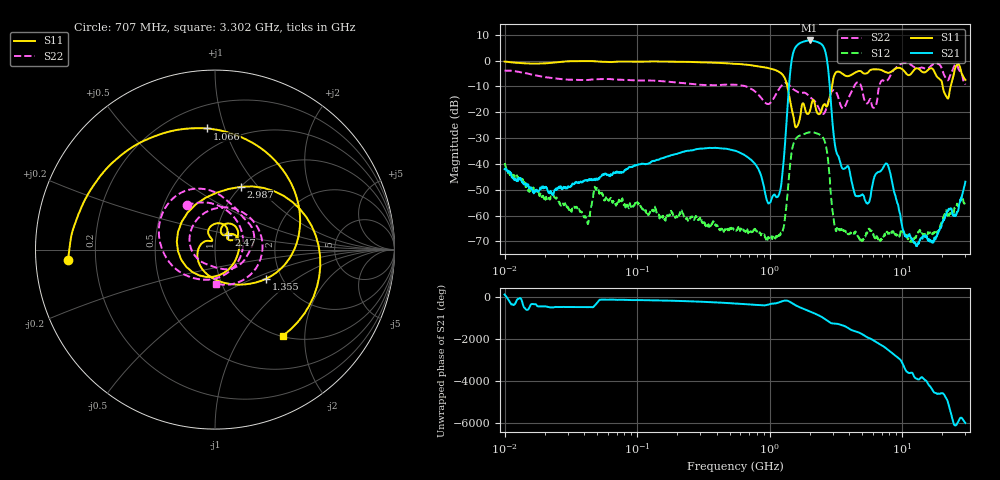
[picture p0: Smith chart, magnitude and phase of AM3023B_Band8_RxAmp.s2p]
# Hz S DB R 50.0
!freq dBS11 angS11 dBS21 angS21 dBS12 angS12 dBS22 angS22
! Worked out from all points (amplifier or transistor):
!   1601 points, 10 MHz to 30 GHz, reference 50 ohm
!   highest |S21| = 7.8 dB at 2.002 GHz (marker M1)
!   |S21| within 3 dB of that: 1.553 GHz to 2.581 GHz (1.028 GHz wide, 49.7 % of centre)
!   unconditionally stable (mu >= 1): start of sweep to end of sweep
!   at 37.85 MHz: K = 3480.71, MAG = -32.6 dB, |S12| = -58.6 dB
!   at 547.7 MHz: K = 11715.56, MAG = -28.5 dB, |S12| = -65.3 dB
!   at 30 GHz: K = 54787.46, MAG = -45.5 dB, |S12| = -56.7 dB
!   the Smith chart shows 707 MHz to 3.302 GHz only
!   S11 on the Smith chart (normalised r, x): 707 MHz: 0.10, -0.04; 1.066 GHz: 0.35, +0.87; 1.355 GHz: 1.66, -0.60; 2.47 GHz: 1.14, +0.19; 2.987 GHz: 1.00, +0.81; 3.302 GHz: 1.02, -1.56
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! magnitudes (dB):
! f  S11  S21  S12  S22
! 10 MHz  -0.4  -42.0  -39.7  -3.9
! 38.04 MHz  -0.2  -47.2  -58.6  -7.5
! 49.35 MHz  -0.3  -45.8  -49.4  -7.2
! 144.7 MHz  -0.4  -38.4  -59.6  -7.9
! 547.7 MHz  -1.3  -34.9  -65.3  -9.4
! 707 MHz  -1.7  -38.0  -66.0  -10.6
! 1.066 GHz  -3.4  -52.2  -68.4  -14.9
! 1.214 GHz  -4.8  -49.2  -66.6  -10.1
! 1.355 GHz  -9.7  -20.2  -53.1  -8.8
! 1.52 GHz  -22.2  3.7  -31.9  -11.3
! 2.002 GHz  -19.8  7.8  -27.8  -14.0
! 2.084 GHz  -16.2  7.7  -27.8  -14.7
! 2.47 GHz  -19.1  6.3  -29.2  -20.3
! 2.987 GHz  -8.5  -24.7  -58.4  -11.6
! 3.302 GHz  -4.3  -37.0  -65.3  -14.4
! 5.446 GHz  -4.9  -55.2  -66.9  -16.6
! 7.926 GHz  -4.7  -41.5  -66.8  -7.0
! 10.33 GHz  -4.0  -66.5  -66.5  -0.9
! 12.69 GHz  -3.1  -71.1  -68.6  -3.0
! 21.67 GHz  -14.1  -59.1  -58.5  -7.3
! 25.95 GHz  -1.6  -58.6  -55.4  -1.6
! 30 GHz  -7.5  -46.9  -56.7  -9.3
